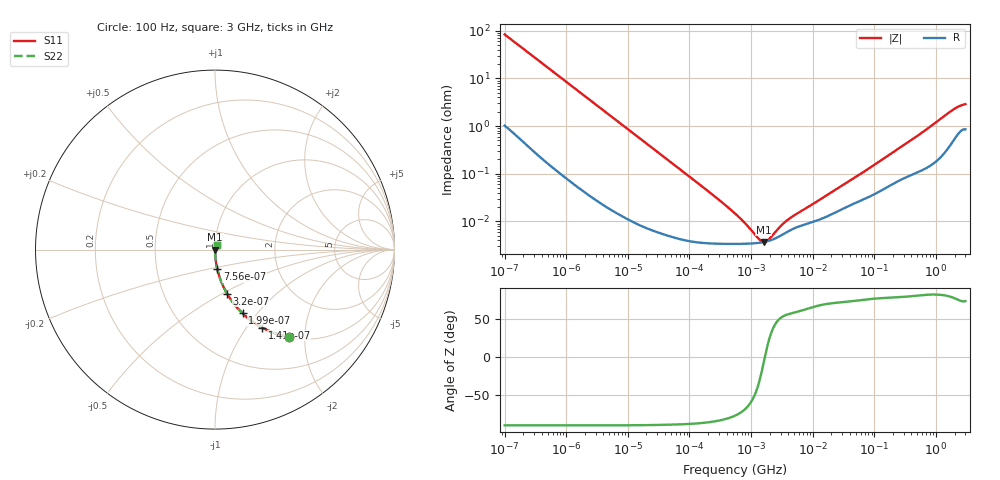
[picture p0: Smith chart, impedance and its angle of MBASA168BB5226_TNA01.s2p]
! MBASA168BB5226_TNA01  S-PARAMETER MODEL  ( Standard Model )
! Model Generated by TAIYO YUDEN Corporation (http://www.ty-top.com)
! Version 2.0
! TAIYO YUDEN Control No. 241120
! Copyright(c) 2012 TAIYO YUDEN CO.,LTD. All Rights Reserved.
! Product Description (link to TY-COMPAS)
! https://ds.yuden.co.jp/TYCOMPAS/or/detail?pn=MBASA168BB5226MTNA01&u=M
! Products Name : Multilayer Ceramic Capacitors
! Characteristics :
!  Capacitance : 22 [uF] , Rated Voltage : 4 [V] , TCC : X5R
!  Case Size : 1.6 x 0.8 / 0.063 x 0.031 [mm/inch] , Thickness : 0.8 / 0.031 [mm/inch]
!  (Conditions: Temperature = 25 [degC] , DC Bias Voltage = 0 [V])
! External Node Assignments :
!  1  o---| |---o  2
! GND o---------o GND
! Frequency Range : 100Hz  -  3GHz  [ 401 STEP ]
# MHZ S RI R 50
! Freq[MHz].  S11 Real  S11 Imag  S21 Real  S21 Imag  S12 Real  S12 Imag  S22 Real  S22 Imag
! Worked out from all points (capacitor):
!   401 points, 100 Hz to 3 GHz, reference 50 ohm
!   read as one part in series: C = 19.1 uF near 109 Hz
!   lowest |Z| = 3.7 mohm at 1.607 MHz (marker M1)
!   series resonance near 1.675 MHz, so ESL is about 470 pH
!   S11 on the Smith chart (normalised r, x): 100 Hz: 1.02, -1.67; 141 Hz: 1.01, -1.18; 199 Hz: 1.01, -0.84; 320 Hz: 1.01, -0.53; 756 Hz: 1.00, -0.22; 3 GHz: 1.02, +0.06
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0.0001  0.4109 -0.4859  0.5891 0.4859  0.5891 0.4859  0.4109 -0.4859
0.000141  0.2623 -0.434  0.7377 0.434  0.7377 0.434  0.2623 -0.434
0.000199  0.1533 -0.3548  0.8467 0.3548  0.8467 0.3548  0.1533 -0.3548
0.00032  0.0669 -0.2448  0.9331 0.2448  0.9331 0.2448  0.0669 -0.2448
0.000471  0.0326 -0.1728  0.9674 0.1728  0.9674 0.1728  0.0326 -0.1728
0.000756  0.0134 -0.1101  0.9866 0.1101  0.9866 0.1101  0.0134 -0.1101
0.001788  0.00269 -0.0473  0.9973 0.0473  0.9973 0.0473  0.00269 -0.0473
0.005476  0.000413 -0.0156  0.9996 0.0156  0.9996 0.0156  0.000413 -0.0156
0.031977  6.47e-05 -0.0027  0.9999 0.0027  0.9999 0.0027  6.47e-05 -0.0027
0.221826  3.45e-05 -0.000386  1 0.000386  1 0.000386  3.45e-05 -0.000386
0.547723  3.36e-05 -0.000142  1 0.000142  1 0.000142  3.36e-05 -0.000142
0.679242  3.37e-05 -0.000107  1 0.000107  1 0.000107  3.37e-05 -0.000107
0.772864  3.38e-05 -8.91e-05  1 8.91e-05  1 8.91e-05  3.38e-05 -8.91e-05
1.6065  3.67e-05 -4.39e-06  1 4.39e-06  1 4.39e-06  3.67e-05 -4.39e-06
3.639519  5.77e-05 8.1e-05  0.9999 -8.1e-05  0.9999 -8.1e-05  5.77e-05 8.1e-05
9.794414  9.61e-05 0.000204  0.9999 -0.000204  0.9999 -0.000204  9.61e-05 0.000204
59.714  0.000272 0.000951  0.9997 -0.000951  0.9997 -0.000951  0.000272 0.000951
175.1444  0.000558 0.00243  0.9994 -0.00243  0.9994 -0.00243  0.000558 0.00243
513.708  0.00112 0.00626  0.9989 -0.00626  0.9989 -0.00626  0.00112 0.00626
1868.531  0.00511 0.021  0.9949 -0.021  0.9949 -0.021  0.00511 0.021
2419.119  0.00798 0.0249  0.992 -0.0249  0.992 -0.0249  0.00798 0.0249
3000  0.00918 0.027  0.9908 -0.027  0.9908 -0.027  0.00918 0.027
